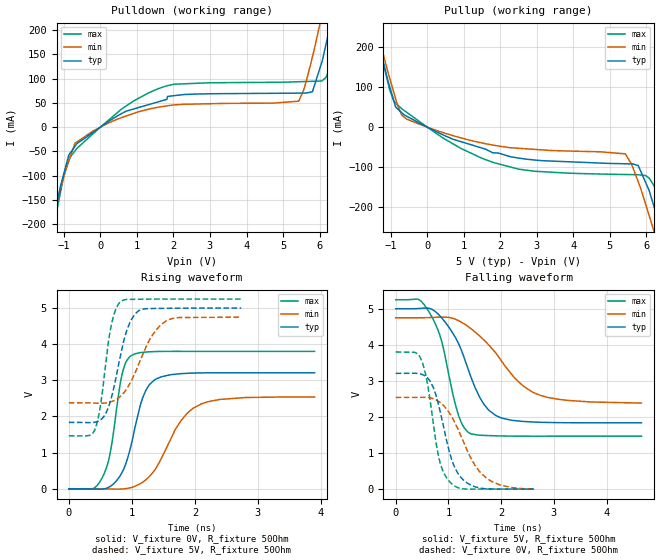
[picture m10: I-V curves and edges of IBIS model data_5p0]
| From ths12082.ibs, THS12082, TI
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|   data_5p0 Model
[Model]   data_5p0
Model_type   Output
Polarity   Non-Inverting
Vmeas = 2.5
Vref = 2.5
Cref = 2pF
Rref = 50
|   typ   min   max
|   (nom PVT)   (fast PVT)   (slow PVT)
C_comp   1.852e-12   1.842e-12   1.903e-12
|ON state : BUFFER OUTPUT TURNED HIGH
|C_comp   1.852e-12   1.842e-12   1.903e-12
|OFF state: BUFFER OUTPUT TURNED LOW
|C_comp   1.650e-12   1.650e-12   1.693e-12
| Where nom  PVT is Nominal Process, 5V, 27C
|   Fast PVT is Strong Process,  5.25V, -55C
|   Slow PVT is Weak Process,   4.75V, 125C
[Voltage Range]   5   4.75   5.25
|Ambient Temperature   25   125   -55
|Junction Temperature
[Temperature Range]   27   125   -55
[Pullup Reference]   5   4.75   5.25
[Pulldown Reference]   0   0   0
[Power Clamp Reference]   5   4.75   5.25
[GND Clamp Reference]   0   0   0
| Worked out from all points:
|   slope of the pulldown table from 0 to 0.75 V, typ, clamps not added: 22.1 ohm
|   slope of the pullup table from 0 to 0.75 V, typ, clamps not added: 23.8 ohm
|   falling waveform, V_fixture 5V, R_fixture 50Ohm: 20-80 % time 559ps typ, 854ps min, 378ps max; typ from 5 V to 1.84 V
|   rising waveform, V_fixture 0V, R_fixture 50Ohm: 20-80 % time 290ps typ, 491ps min, 202ps max; typ from 0 V to 3.21 V
|   rising waveform, V_fixture 5V, R_fixture 50Ohm: 20-80 % time 250ps typ, 388ps min, 176ps max; typ from 1.84 V to 5 V
|   falling waveform, V_fixture 0V, R_fixture 50Ohm: 20-80 % time 337ps typ, 526ps min, 251ps max; typ from 3.21 V to 0 V
[Pulldown]
|   Voltage   I(typ)   I(min)   I(max)
-5V       -1.618A    -1.482A    -1.792A
-1.302V   -192.5mA   -190.7mA   -214.4mA
-997.5mV  -95.28mA   -101.9mA   -98.24mA
-693.5mV  -39.39mA   -33.02mA   -48.8mA
924mV     37.72mA    28.66mA    54.61mA
2.026V    64.97mA    45.8mA     88.52mA
5.425V    70.14mA    53.51mA    93.64mA
5.805V    72.99mA    144.9mA    94.52mA
6.053V    131.9mA    227.6mA    95.09mA
6.3V      212.3mA    311mA      131.6mA
6.525V    291.6mA    387.1mA    210.5mA
10V       1.651A     1.701A     1.602A
[Pullup]
|   Voltage   I(typ)   I(min)   I(max)
-5V       1.699A     1.64A      1.754A
-2.627V   724.6mA    714.2mA    756.1mA
-1.31V    202.4mA    220.3mA    202.5mA
-1.034V   103.2mA    124.8mA    95.5mA
-698.3mV  36.05mA    30.47mA    46.07mA
251.7mV   -11.59mA   -8.176mA   -15.95mA
2.499V    -77.51mA   -52.94mA   -105.3mA
5.415V    -91.78mA   -66.9mA    -118.7mA
5.775V    -96.31mA   -136.8mA   -119.3mA
6.216V    -201.9mA   -263.3mA   -148.4mA
6.525V    -301.4mA   -354.2mA   -252.5mA
10V       -1.621A    -1.569A    -1.695A
[Ramp]
R_load = 50
|   typ   min   max
dV/dt_r   1.92517/2.89065e-10   1.52418/4.88527e-10   2.28117/2.01302e-10
dV/dt_f   1.89786/5.58448e-10   1.4231/8.5709e-10   2.27022/3.76094e-10
[Falling Waveform]
V_fixture = 5V
V_fixture_min = 4.75V
V_fixture_max = 5.25V
R_fixture = 50Ohm
|   Time   V(typ)   V(min)   V(max)
0s        5V         4.75V      5.25V
434ps     5.007V     4.749V     5.259V
672ps     4.995V     4.757V     4.81V
880ps     4.733V     4.769V     4.056V
1.19ns    4.038V     4.672V     2.049V
1.418ns   3.141V     4.457V     1.535V
1.672ns   2.355V     4.135V     1.489V
1.892ns   2.047V     3.783V     1.477V
2.644ns   1.858V     2.656V     1.466V
4.66ns    1.837V     2.385V     1.466V
[Rising Waveform]
V_fixture = 0V
V_fixture_min = 0V
V_fixture_max = 0V
R_fixture = 50Ohm
|   Time   V(typ)   V(min)   V(max)
0s        1.848nV    2.664nV    1.571nV
552ps     -5.002mV   -2.71mV    382.9mV
660ps     68.81mV    -6.155mV   1.026V
842ps     445.1mV    -6.535mV   3.145V
992ps     1.234V     35.5mV     3.686V
1.218ns   2.707V     243mV      3.783V
1.46ns    3.093V     810.6mV    3.8V
1.776ns   3.185V     1.875V     3.803V
2.102ns   3.207V     2.347V     3.802V
3.899ns   3.209V     2.54V      3.802V
[Rising Waveform]
V_fixture = 5V
V_fixture_min = 4.75V
V_fixture_max = 5.25V
R_fixture = 50Ohm
|   Time   V(typ)   V(min)   V(max)
0s        1.837V     2.378V     1.466V
418ps     1.844V     2.371V     1.655V
502ps     1.905V     2.367V     2.304V
680ps     2.55V      2.413V     4.577V
838ps     3.832V     2.588V     5.202V
936ps     4.46V      2.814V     5.24V
1.058ns   4.85V      3.233V     5.243V
1.308ns   4.987V     4.203V     5.248V
1.55ns    4.994V     4.651V     5.25V
2.736ns   5V         4.75V      5.25V
[Falling Waveform]
V_fixture = 0V
V_fixture_min = 0V
V_fixture_max = 0V
R_fixture = 50Ohm
|   Time   V(typ)   V(min)   V(max)
0s        3.209V     2.54V      3.802V
478ps     3.191V     2.544V     3.608V
600ps     3.085V     2.539V     2.938V
716ps     2.805V     2.503V     1.792V
840ps     2.174V     2.403V     742.1mV
1.054ns   852.2mV    2.026V     157.2mV
1.298ns   232.6mV    1.27V      3.84mV
1.508ns   61.13mV    649.2mV    -12.99uV
1.716ns   6.151mV    311.4mV    465.4uV
2.624ns   424.6uV    1.621mV    145.9uV
